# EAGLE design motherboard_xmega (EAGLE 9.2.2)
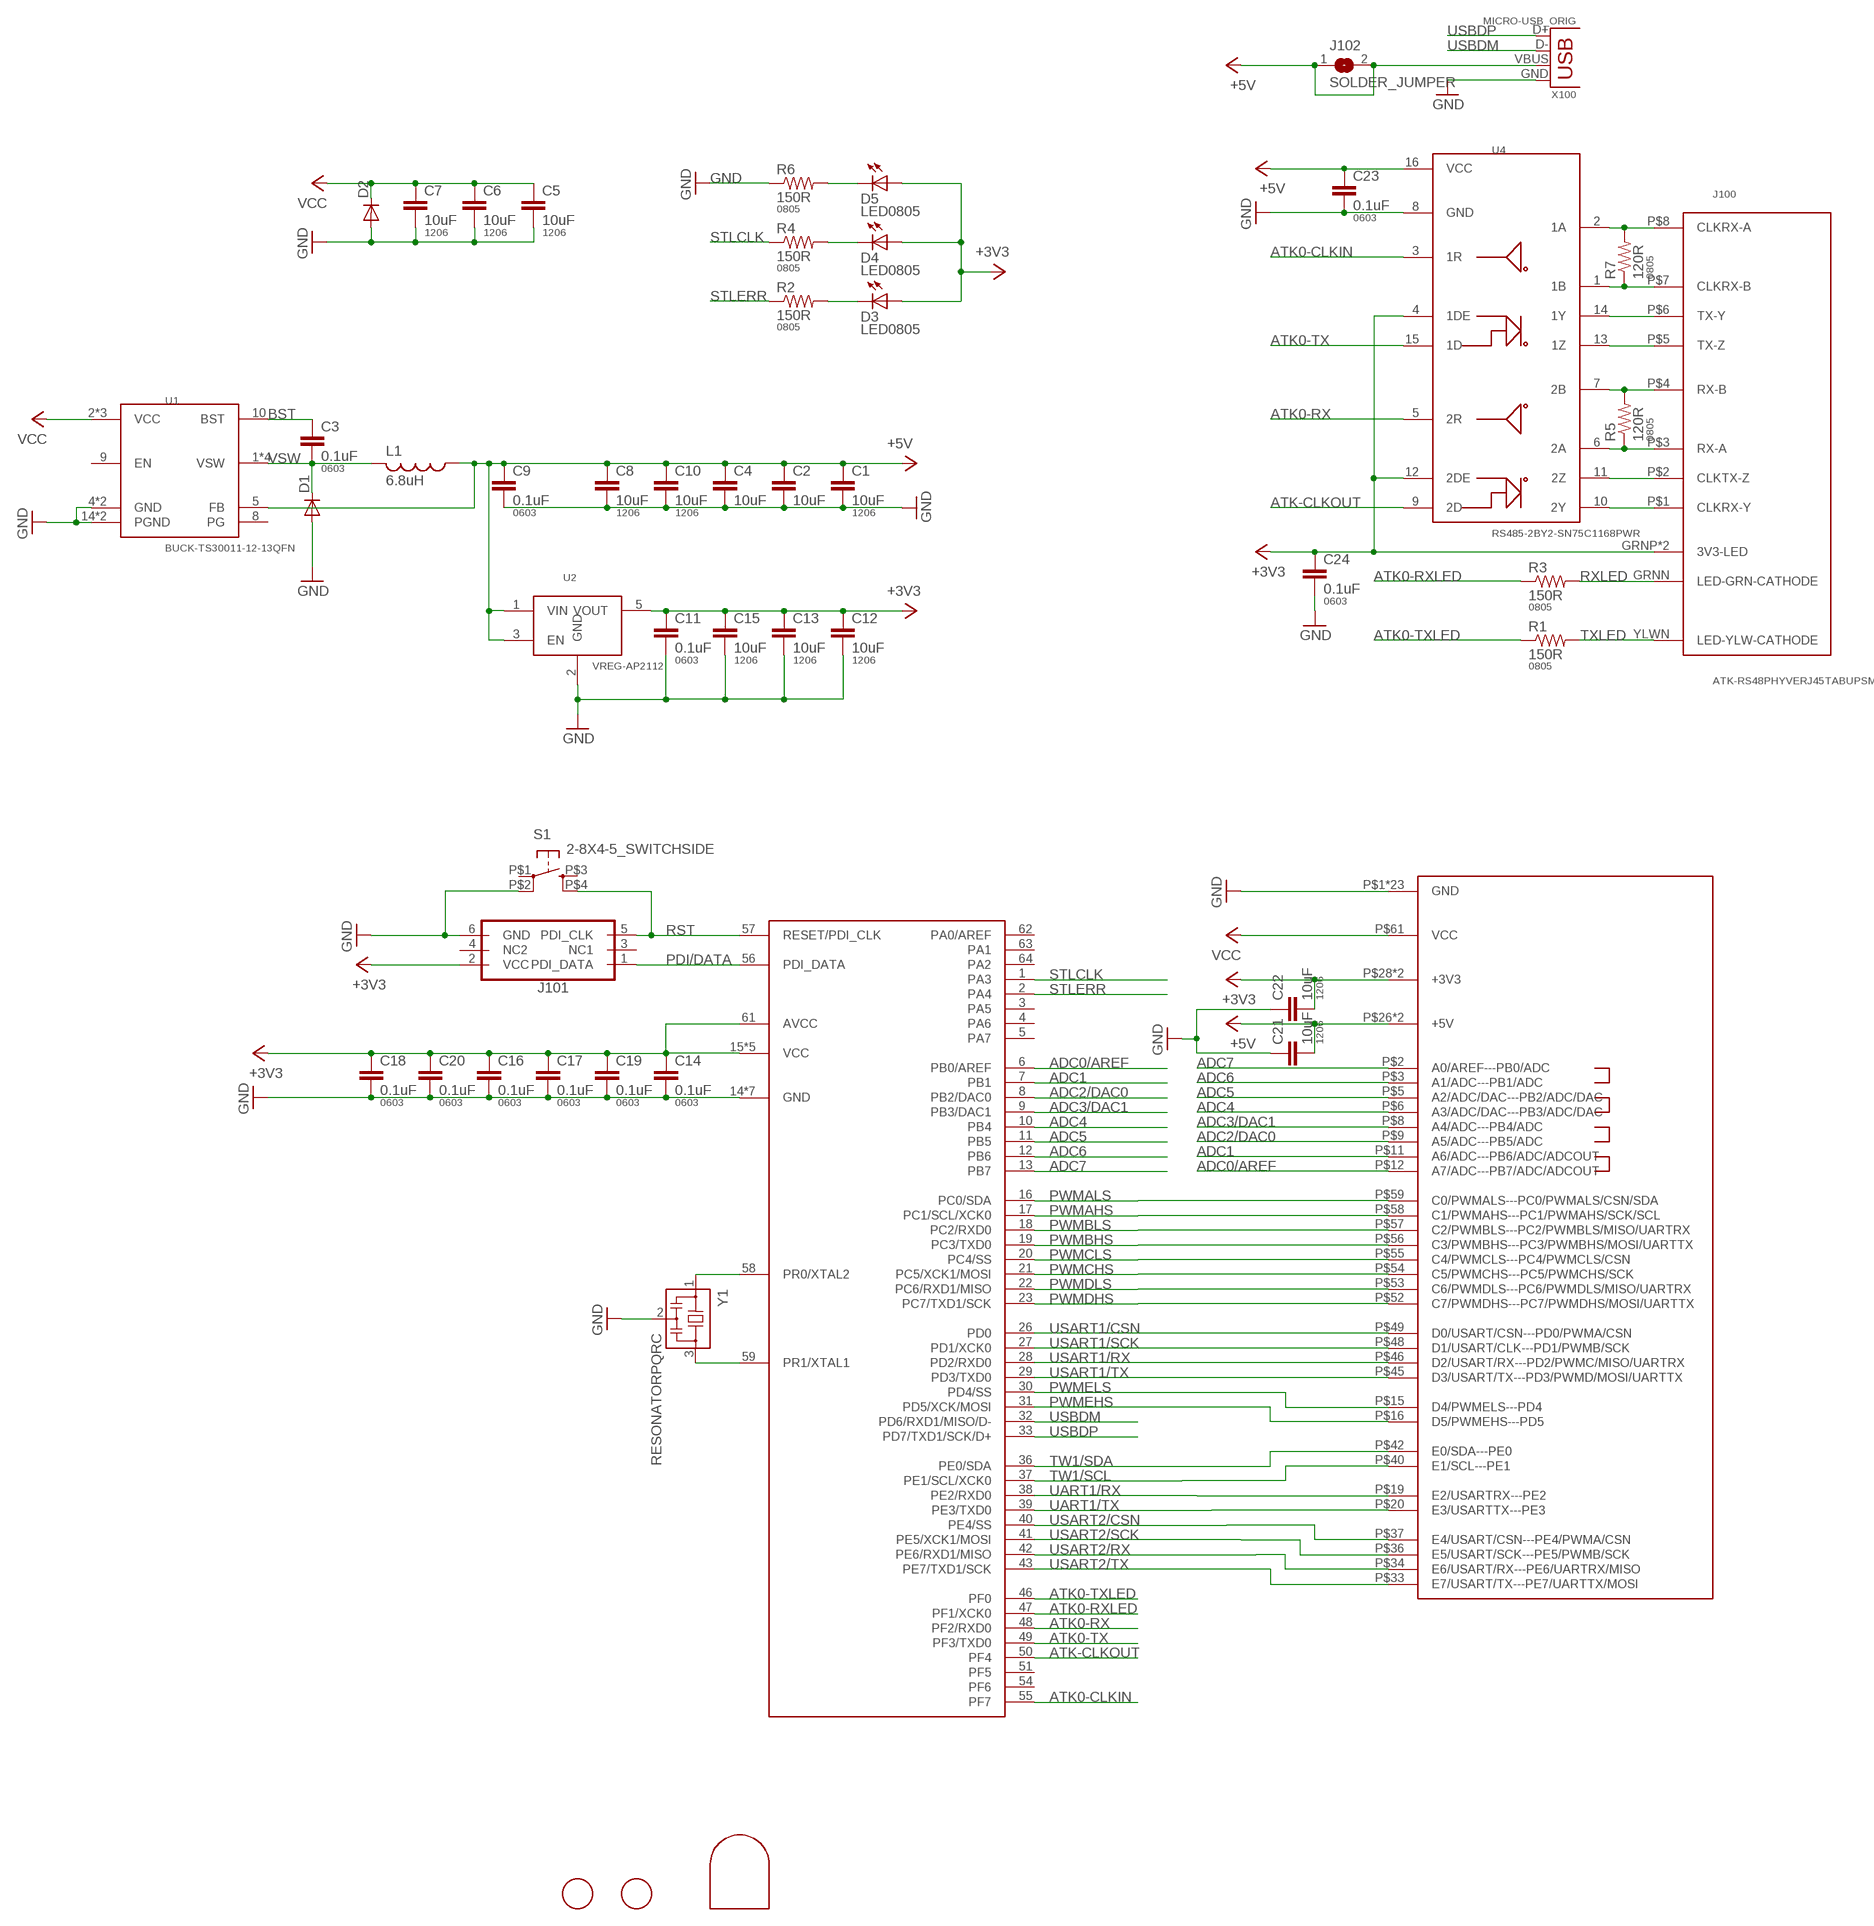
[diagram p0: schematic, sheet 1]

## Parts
C1  10uF  CAP1206  [1206]
C2  10uF  CAP1206  [1206]
C3  0.1uF  CAP0603-CAP  [0603-CAP]
C4  10uF  CAP1206  [1206]
C5  10uF  CAP1206  [1206]
C6  10uF  CAP1206  [1206]
C7  10uF  CAP1206  [1206]
C8  10uF  CAP1206  [1206]
C9  0.1uF  CAP0603-CAP  [0603-CAP]
C10  10uF  CAP1206  [1206]
C11  0.1uF  CAP0603-CAP  [0603-CAP]
C12  10uF  CAP1206  [1206]
C13  10uF  CAP1206  [1206]
C14  0.1uF  CAP0603-CAP  [0603-CAP]
C15  10uF  CAP1206  [1206]
C16  0.1uF  CAP0603-CAP  [0603-CAP]
C17  0.1uF  CAP0603-CAP  [0603-CAP]
C18  0.1uF  CAP0603-CAP  [0603-CAP]
C19  0.1uF  CAP0603-CAP  [0603-CAP]
C20  0.1uF  CAP0603-CAP  [0603-CAP]
C21  10uF  CAP1206  [1206]
C22  10uF  CAP1206  [1206]
C23  0.1uF  CAP0603-CAP  [0603-CAP]
C24  0.1uF  CAP0603-CAP  [0603-CAP]
D1  DIODESOD123HE  [SOD-123HE]
D2  DIODESMA403D  [SMA-403D]
D3  LED0805  [LED0805]
D4  LED0805  [LED0805]
D5  LED0805  [LED0805]
J1  FIDUCIALRCT  [FIDUCIAL_RECT_1MM]
J2  FIDUCIALRCT  [FIDUCIAL_RECT_1MM]
J100  ATK-RS48PHYVERJ45TABUPSMD  [RJ45-LED-SMD-RJWURTH-634008137521]
J101  PDITHRU  [PDI_2X3_THRU]
J102  SOLDER_JUMPER  [SJFAB]
L1  6.8uH  INDUCTOR  [NRS5020T4R7MMGJ]
MP100  JRTOMBSTONE  [JRTOMBSTONE]
R1  150R  RESISTOR0805-RES  [0805]
R2  150R  RESISTOR0805-RES  [0805]
R3  150R  RESISTOR0805-RES  [0805]
R4  150R  RESISTOR0805-RES  [0805]
R5  120R  RESISTOR0805-RES  [0805]
R6  150R  RESISTOR0805-RES  [0805]
R7  120R  RESISTOR0805-RES  [0805]
S1  2-8X4-5_SWITCHSIDE  [TACT-SWITCH-SIDE]
U1  BUCK-TS30011-12-13QFN  [QFN16-3X3-TI-RTE]
U2  VREG-AP2112  [SOT23-5]
U3  ATXMEGA_A3UQFN  [QFN-64-9X9MM]
U4  RS485-2BY2-SN75C1168PWR  [TSSOP16]
U$100  ATK-BFPPFX8-MOTHER  [ATK-BFPP-BOTTOM-FX8-60]
X100  MICRO-USB_ORIG  [DX4R005HJ5]
Y1  RESONATORPQRC  [RES_PRQC]

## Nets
+3V3: C11.1 C12.1 C13.1 C14.1 C15.1 C16.1 C17.1 C18.1 C19.1 C20.1 C22.2 C24.1 D3.1(A) D4.1(A) D5.1(A) J100.GRNP(3V3-LED) J100.YLWP(3V3-LED) J101.2(VCC) U2.5(VOUT) U3.15(VCC) U3.25(VCC) U3.35(VCC) U3.45(VCC) U3.53(VCC) U3.61(AVCC) U4.4(1DE) U4.12(2DE) U$100.P$28(+3V3) U$100.P$29(+3V3)
+5V: C1.1 C2.1 C4.1 C8.1 C9.1 C10.1 C21.2 C23.1 J102.1 J102.2 L1.1 U1.5(FB) U2.1(VIN) U2.3(EN) U4.16(VCC) U$100.P$26(+5V) U$100.P$27(+5V) X100.VBUS
ADC0/AREF: U3.6(PB0/AREF) U$100.P$12(A7/ADC---PB7/ADC/ADCOUT)
ADC1: U3.7(PB1) U$100.P$11(A6/ADC---PB6/ADC/ADCOUT)
ADC2/DAC0: U3.8(PB2/DAC0) U$100.P$9(A5/ADC---PB5/ADC)
ADC3/DAC1: U3.9(PB3/DAC1) U$100.P$8(A4/ADC---PB4/ADC)
ADC4: U3.10(PB4) U$100.P$6(A3/ADC/DAC---PB3/ADC/DAC)
ADC5: U3.11(PB5) U$100.P$5(A2/ADC/DAC---PB2/ADC/DAC)
ADC6: U3.12(PB6) U$100.P$3(A1/ADC---PB1/ADC)
ADC7: U3.13(PB7) U$100.P$2(A0/AREF---PB0/ADC)
ATK0-CLKIN: U3.55(PF7) U4.3(1R)
ATK0-RX: U3.48(PF2/RXD0) U4.5(2R)
ATK0-RXLED: R3.1 U3.47(PF1/XCK0)
ATK0-TX: U3.49(PF3/TXD0) U4.15(1D)
ATK0-TXLED: R1.1 U3.46(PF0)
ATK-CLKOUT: U3.50(PF4) U4.9(2D)
BST: C3.1 U1.10(BST)
GND: C1.2 C2.2 C4.2 C5.2 C6.2 C7.2 C8.2 C9.2 C10.2 C11.2 C12.2 C13.2 C14.2 C15.2 C16.2 C17.2 C18.2 C19.2 C20.2 C21.1 C22.1 C23.2 C24.2 D1.P$2(A) D2.P$2(A) J101.6(GND) R6.1 S1.P$2(P1) U1.4(GND) U1.14(PGND) U1.15(PGND) U1.TH(GND) U2.2(GND) U3.14(GND) U3.24(GND) U3.34(GND) U3.44(GND) U3.52(GND) U3.60(GND) U3.P$1(GND) U4.8(GND) U$100.P$1(GND) U$100.P$4(GND) U$100.P$7(GND) U$100.P$10(GND) U$100.P$13(GND) U$100.P$14(GND) U$100.P$17(GND) U$100.P$18(GND) U$100.P$21(GND) U$100.P$30(GND) U$100.P$31(GND) U$100.P$32(GND) U$100.P$35(GND) U$100.P$38(GND) U$100.P$39(GND) U$100.P$41(GND) U$100.P$43(GND) U$100.P$44(GND) U$100.P$47(GND) U$100.P$50(GND) U$100.P$51(GND) U$100.P$60(GND) U$100.P$62(GND) X100.GND Y1.2
N$1: U3.58(PR0/XTAL2) Y1.1
N$2: U3.59(PR1/XTAL1) Y1.3
N$8: J100.P$8(CLKRX-A) R7.2 U4.2(1A)
N$9: D5.2(C) R6.2
N$10: D4.2(C) R4.2
N$11: D3.2(C) R2.2
N$12: J100.P$7(CLKRX-B) R7.1 U4.1(1B)
N$13: J100.P$6(TX-Y) U4.14(1Y)
N$14: J100.P$5(TX-Z) U4.13(1Z)
N$15: J100.P$4(RX-B) R5.2 U4.7(2B)
N$16: J100.P$3(RX-A) R5.1 U4.6(2A)
N$17: J100.P$2(CLKTX-Z) U4.11(2Z)
N$18: J100.P$1(CLKRX-Y) U4.10(2Y)
PDI/DATA: J101.1(PDI_DATA) U3.56(PDI_DATA)
PWMAHS: U3.17(PC1/SCL/XCK0) U$100.P$58(C1/PWMAHS---PC1/PWMAHS/SCK/SCL)
PWMALS: U3.16(PC0/SDA) U$100.P$59(C0/PWMALS---PC0/PWMALS/CSN/SDA)
PWMBHS: U3.19(PC3/TXD0) U$100.P$56(C3/PWMBHS---PC3/PWMBHS/MOSI/UARTTX)
PWMBLS: U3.18(PC2/RXD0) U$100.P$57(C2/PWMBLS---PC2/PWMBLS/MISO/UARTRX)
PWMCHS: U3.21(PC5/XCK1/MOSI) U$100.P$54(C5/PWMCHS---PC5/PWMCHS/SCK)
PWMCLS: U3.20(PC4/SS) U$100.P$55(C4/PWMCLS---PC4/PWMCLS/CSN)
PWMDHS: U3.23(PC7/TXD1/SCK) U$100.P$52(C7/PWMDHS---PC7/PWMDHS/MOSI/UARTTX)
PWMDLS: U3.22(PC6/RXD1/MISO) U$100.P$53(C6/PWMDLS---PC6/PWMDLS/MISO/UARTRX)
PWMEHS: U3.31(PD5/XCK/MOSI) U$100.P$16(D5/PWMEHS---PD5)
PWMELS: U3.30(PD4/SS) U$100.P$15(D4/PWMELS---PD4)
RST: J101.5(PDI_CLK) S1.P$4(S1) U3.57(RESET/PDI_CLK)
RXLED: J100.GRNN(LED-GRN-CATHODE) R3.2
STLCLK: R4.1 U3.1(PA3)
STLERR: R2.1 U3.2(PA4)
TW1/SCL: U3.37(PE1/SCL/XCK0) U$100.P$40(E1/SCL---PE1)
TW1/SDA: U3.36(PE0/SDA) U$100.P$42(E0/SDA---PE0)
TXLED: J100.YLWN(LED-YLW-CATHODE) R1.2
UART1/RX: U3.38(PE2/RXD0) U$100.P$19(E2/USARTRX---PE2)
UART1/TX: U3.39(PE3/TXD0) U$100.P$20(E3/USARTTX---PE3)
USART1/CSN: U3.26(PD0) U$100.P$49(D0/USART/CSN---PD0/PWMA/CSN)
USART1/RX: U3.28(PD2/RXD0) U$100.P$46(D2/USART/RX---PD2/PWMC/MISO/UARTRX)
USART1/SCK: U3.27(PD1/XCK0) U$100.P$48(D1/USART/CLK---PD1/PWMB/SCK)
USART1/TX: U3.29(PD3/TXD0) U$100.P$45(D3/USART/TX---PD3/PWMD/MOSI/UARTTX)
USART2/CSN: U3.40(PE4/SS) U$100.P$37(E4/USART/CSN---PE4/PWMA/CSN)
USART2/RX: U3.42(PE6/RXD1/MISO) U$100.P$34(E6/USART/RX---PE6/UARTRX/MISO)
USART2/SCK: U3.41(PE5/XCK1/MOSI) U$100.P$36(E5/USART/SCK---PE5/PWMB/SCK)
USART2/TX: U3.43(PE7/TXD1/SCK) U$100.P$33(E7/USART/TX---PE7/UARTTX/MOSI)
USBDM: U3.32(PD6/RXD1/MISO/D-) X100.D-
USBDP: U3.33(PD7/TXD1/SCK/D+) X100.D+
VCC: C5.1 C6.1 C7.1 D2.P$1(C) U1.2(VCC) U1.3(VCC) U1.11(VCC) U$100.P$61(VCC)
VSW: C3.2 D1.P$1(C) L1.2 U1.1(VSW) U1.12(VSW) U1.13(VSW) U1.16(VSW)
Unconnected: J101.3(NC1) J101.4(NC2) S1.P$1(P) S1.P$3(S) U1.8(PG) U1.9(EN) U3.3(PA5) U3.4(PA6) U3.5(PA7) U3.51(PF5) U3.54(PF6) U3.62(PA0/AREF) U3.63(PA1) U3.64(PA2)

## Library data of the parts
C1 C2 C4-C8 C10 C12 C13 C15 C21 C22 = passives:CAP: Capacitor; PACKAGE: 1206
C3 C9 C11 C14 C16-C20 C23 C24 = passives:CAP: Capacitor; PACKAGE: 0603
D1 D2 = passives:DIODE: DIODE
D3-D5 = lights:LED: LED
J1 J2 = connector:FIDUCIAL: For use by pick and place machines to calibrate the vision/machine, 1mm
J100 = connector:ATK-RS48PHYVE
J101 = microcontrollers:PDI: Multi connection point. Often used as Generic Header-pin footprint for 0.1 inch spaced/style header connections You can populate with any combo of single row headers, but if you'd like an exact match, check these: Header - 2x3 (Male, 0.1") (PRT-12807) Header - 2x3 (Female, 0.1") (PRT-13010) 2x3 Pin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
J102 = connector:SOLDER_JUMPER
L1 = power:INDUCTOR
MP100 = connector:JRTOMBSTONE
R1-R7 = borkedlabs-passives:RESISTOR: Resistor; PACKAGE: 0805
S1 = passives:2-8X4-5_SWITCH
U1 = power:BUCK-TS30011-12-13
U2 = power:VREG-AP2112
U3 = microcontrollers:ATXMEGA_A3U
U4 = comm:RS485-2BY2-SN75C1168PWR
U$100 = connector:ATK-BFPP
X100 = connector:MICRO-USB: SMD micro USB connector as found in the fablab inventory. Three footprint variants included: original, as described by manufacturer's datasheet for milling with the 1/100" bit for milling with the 1/64" bit Made by Zaerc.
Y1 = passives:RESONATOR

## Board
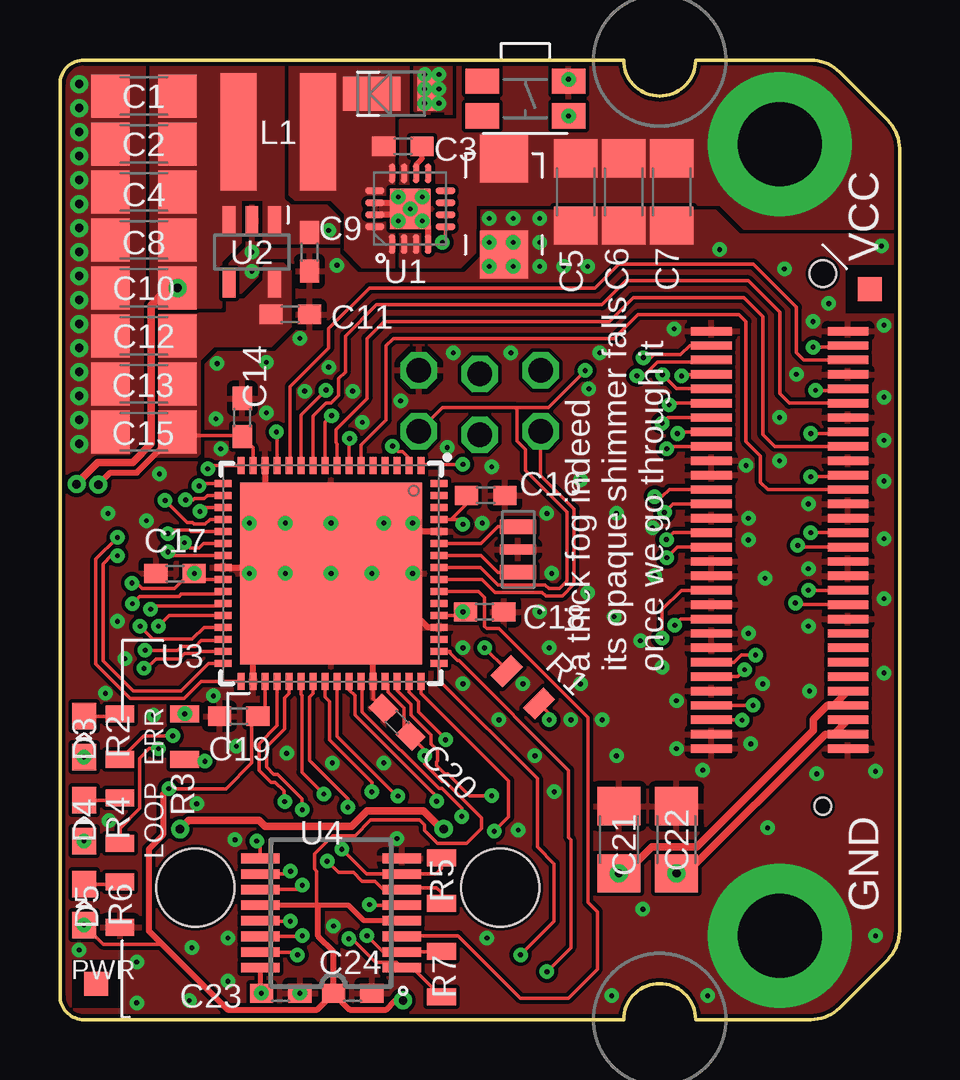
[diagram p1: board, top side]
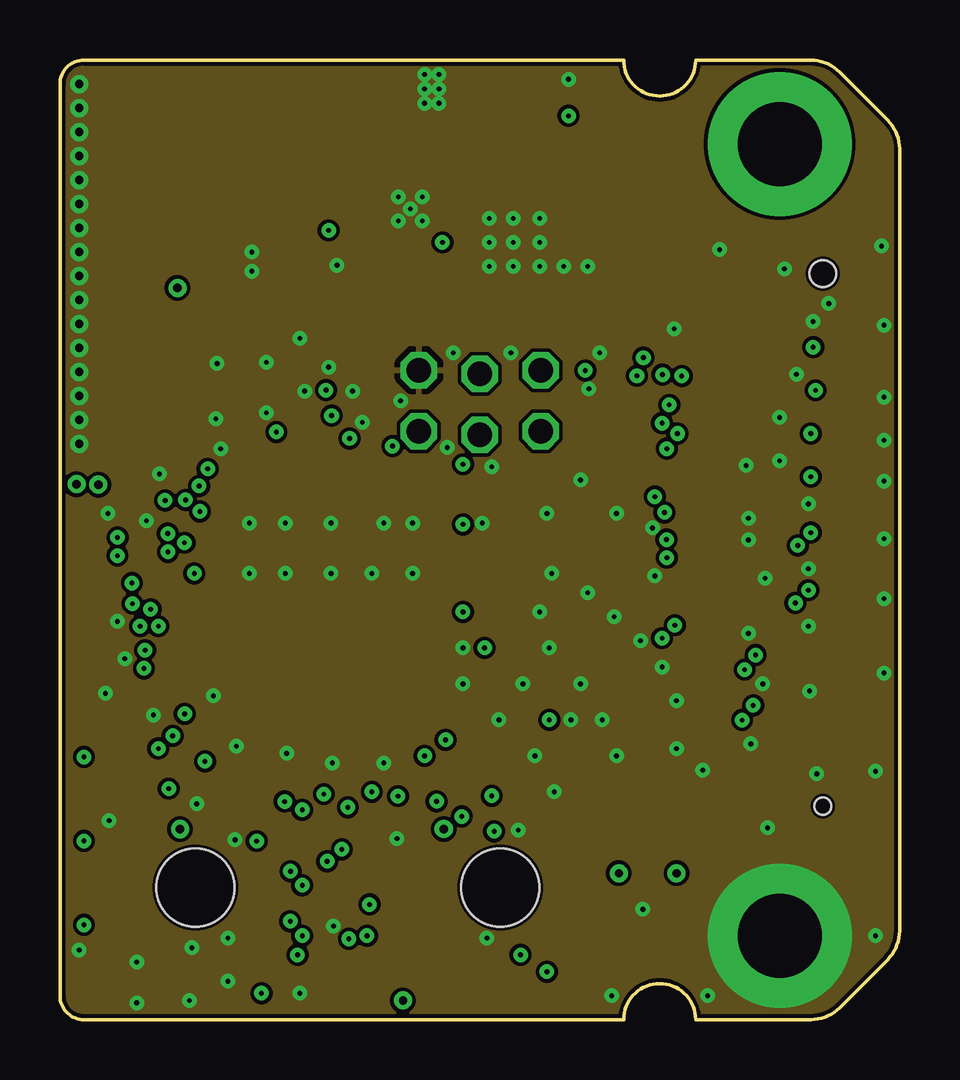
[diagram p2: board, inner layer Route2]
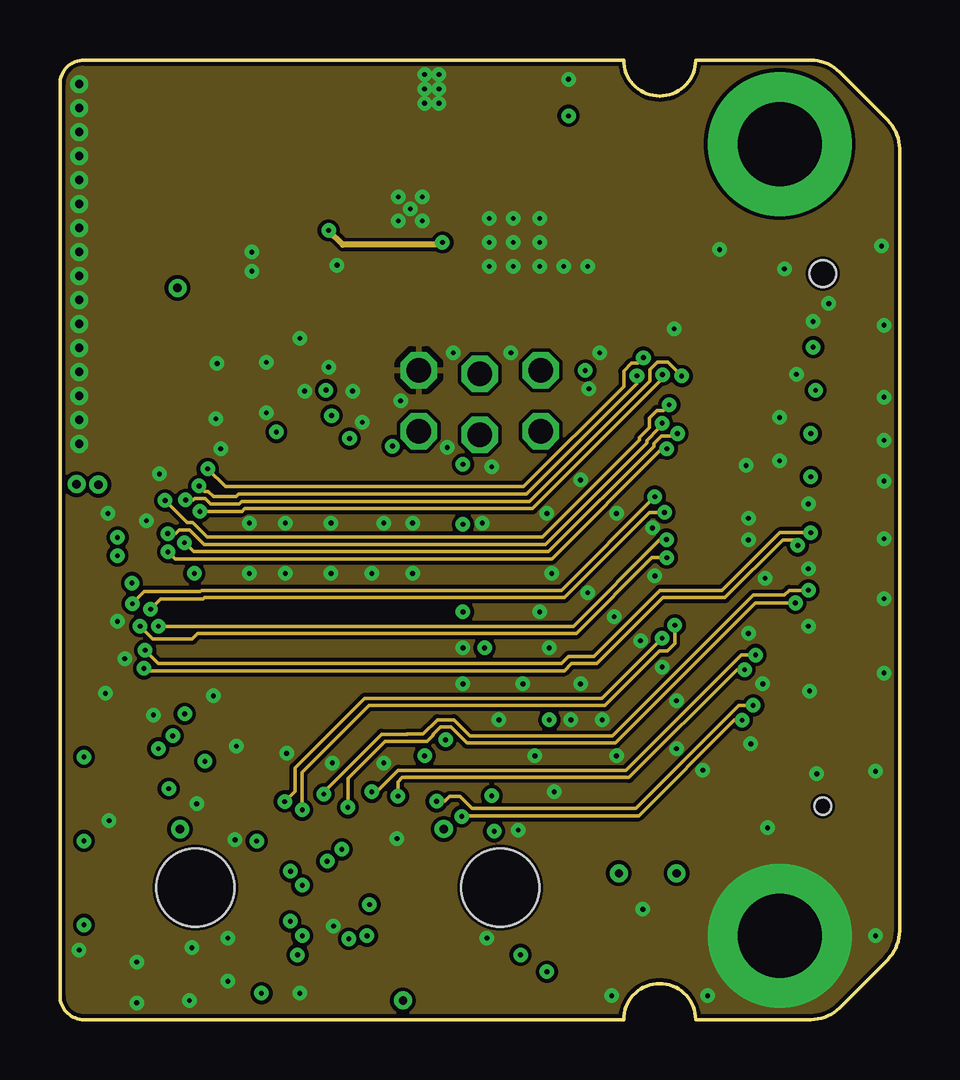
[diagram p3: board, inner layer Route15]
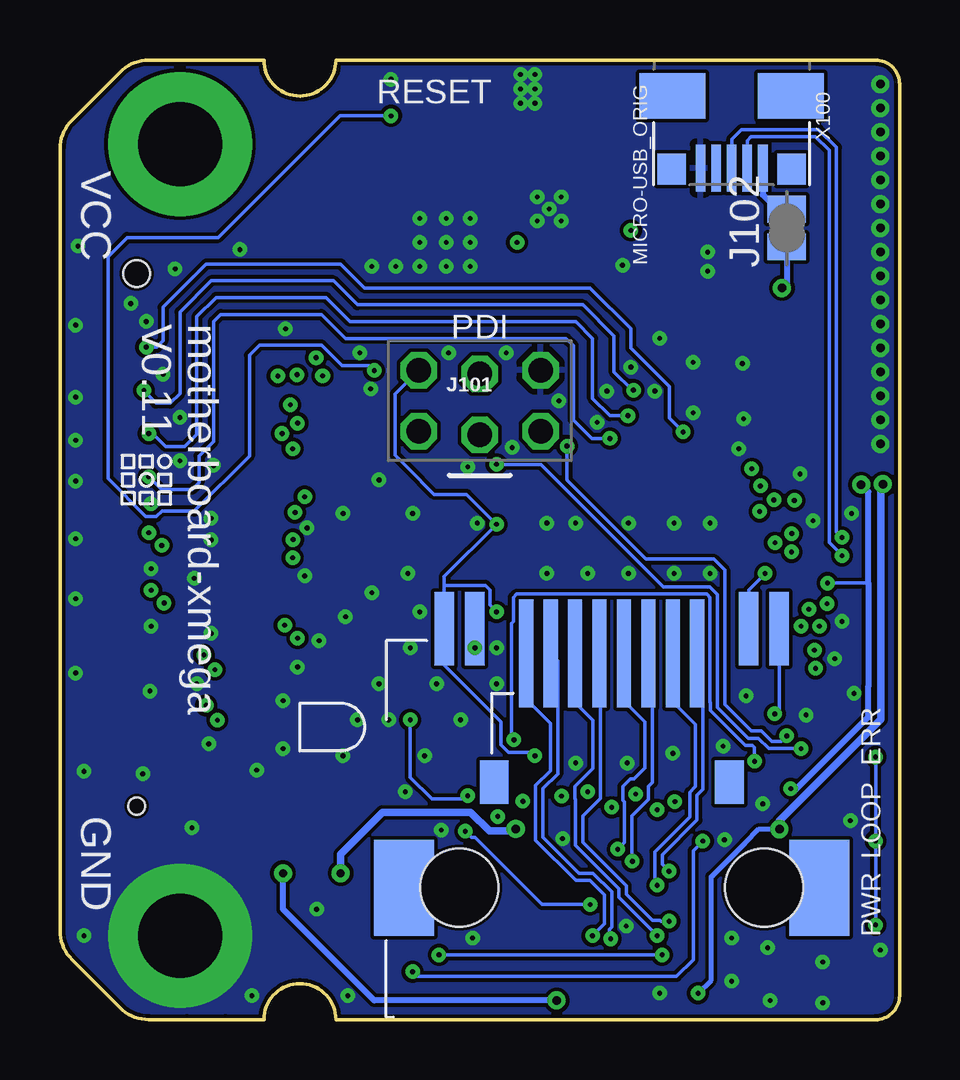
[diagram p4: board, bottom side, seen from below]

Size 35 x 40.01 mm. Coordinates in mm from the lower left corner, seen from the top.
Outline: 23.5,40 arc90 25,38.5 arc90 26.5,40 arc0 31.3,40 arc-45 32.5,39.5 34.5,37.5 arc-45 35,36.3 35,3.7 arc-45 34.5,2.5 32.5,0.5 arc-45 31.3,0 arc0 26.5,0 arc90 25,1.5 arc90 23.5,0 1,0 arc-90 0,1 0,39 arc-90 1,40 23.5,40
Copper layers (1+2*15+16): Top 0.035mm / dielectric 0.3mm / Route2 0.035mm / dielectric 0.3mm / Route15 0.035mm / dielectric 0.3mm / Bottom 0.035mm
Design rules "default *": minimum track width 6mil, minimum drill 0.2mm, track to track 6mil, track to pad 6mil, pad to pad 6mil, via to via 6mil, smd to smd 6mil, copper to edge 6mil, drill to drill 6mil, minimum pad ring 10mil, minimum via ring 8mil, stop-mask expansion 4mil, vias tented up to drill 25mil, thermal gap 10mil

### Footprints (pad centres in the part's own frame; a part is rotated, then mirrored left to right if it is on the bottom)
1206 = smd 1.6 x 1.8: 1 -1.4,0; 2 1.4,0
0603-CAP = smd 0.96 x 0.8: 1 -0.8,0; 2 0.8,0
SOD-123HE = smd 2.4 x 1.4: P$1 0.8,0 | smd 0.9 x 1.4: P$2 -1.55,0
SMA-403D = smd 2 x 2: P$1 -2,0; P$2 2,0
LED0805 = smd 1.1 x 1: 1 -0.85,0; 2 0.85,0
FIDUCIAL_RECT_1MM = smd 1 x 1: P$1 0,0
RJ45-LED-SMD-RJWURTH-634008137521 = smd 0.8 x 3.05: GRNN 6.98,10.8; GRNP 5.71,10.8; YLWN -5.71,10.8; YLWP -6.98,10.8 | smd 0.6 x 4.5: P$1 3.57,9.76; P$2 2.55,9.76; P$3 1.53,9.76; P$4 0.51,9.76; P$5 -0.51,9.76; P$6 -1.53,9.76; P$7 -2.55,9.76; P$8 -3.57,9.76 | smd 1.2 x 1.8: P$9 -4.9,4.4; P$10 4.9,4.4 | smd 2.5 x 4: P$13 -8.65,0; P$14 8.65,0 | hole 3.25: -6.35,0; 6.35,0
PDI_2X3_THRU = drill 1.016 octagon: 1 -2.54,-1.27; 2 -2.54,1.27; 3 0,-1.42; 4 0,1.12; 5 2.54,-1.27; 6 2.54,1.27
SJFAB = smd 1.118 x 1.6: 1 -0.787,0; 2 0.787,0
NRS5020T4R7MMGJ = smd 4.9 x 1.5: 1 0,1.65; 2 0,-1.65
0805 = smd 0.7 x 1.2: 1 -0.95,0; 2 0.95,0
TACT-SWITCH-SIDE = smd 1.4 x 1.05: P$1 -1.8,0.725; P$2 1.8,0.725; P$3 -1.8,-0.725; P$4 1.8,-0.725
QFN16-3X3-TI-RTE = smd 0.8 x 0.275: 1 -1.475,0.75; 2 -1.475,0.25; 3 -1.475,-0.25; 4 -1.475,-0.75; 9 1.475,-0.75; 10 1.475,-0.25; 11 1.475,0.25; 12 1.475,0.75 | smd 0.275 x 0.8: 5 -0.75,-1.475; 6 -0.25,-1.475; 7 0.25,-1.475; 8 0.75,-1.475; 13 0.75,1.475; 14 0.25,1.475; 15 -0.25,1.475; 16 -0.75,1.475 | smd 1.7 x 1.7: TH 0,0
SOT23-5 = smd 0.533 x 1.194: 1 -0.95,-1.306; 2 0,-1.306; 3 0.95,-1.306; 4 0.95,1.306; 5 -0.95,1.306
QFN-64-9X9MM = smd 0.7 x 0.275: 1 -4.5,3.75; 2 -4.5,3.25; 3 -4.5,2.75; 4 -4.5,2.25; 5 -4.5,1.75; 6 -4.5,1.25; 7 -4.5,0.75; 8 -4.5,0.25; 9 -4.5,-0.25; 10 -4.5,-0.75; 11 -4.5,-1.25; 12 -4.5,-1.75; 13 -4.5,-2.25; 14 -4.5,-2.75; 15 -4.5,-3.25; 16 -4.5,-3.75; 33 4.5,-3.75; 34 4.5,-3.25; 35 4.5,-2.75; 36 4.5,-2.25; 37 4.5,-1.75; 38 4.5,-1.25; 39 4.5,-0.75; 40 4.5,-0.25; 41 4.5,0.25; 42 4.5,0.75; 43 4.5,1.25; 44 4.5,1.75; 45 4.5,2.25; 46 4.5,2.75; 47 4.5,3.25; 48 4.5,3.75 | smd 0.275 x 0.7: 17 -3.75,-4.5; 18 -3.25,-4.5; 19 -2.75,-4.5; 20 -2.25,-4.5; 21 -1.75,-4.5; 22 -1.25,-4.5; 23 -0.75,-4.5; 24 -0.25,-4.5; 25 0.25,-4.5; 26 0.75,-4.5; 27 1.25,-4.5; 28 1.75,-4.5; 29 2.25,-4.5; 30 2.75,-4.5; 31 3.25,-4.5; 32 3.75,-4.5; 49 3.75,4.5; 50 3.25,4.5; 51 2.75,4.5; 52 2.25,4.5; 53 1.75,4.5; 54 1.25,4.5; 55 0.75,4.5; 56 0.25,4.5; 57 -0.25,4.5; 58 -0.75,4.5; 59 -1.25,4.5; 60 -1.75,4.5; 61 -2.25,4.5; 62 -2.75,4.5; 63 -3.25,4.5; 64 -3.75,4.5 | smd 7.6 x 7.6: P$1 0,0
TSSOP16 = smd 0.4 x 1.6: 1 -2.225,-2.85; 2 -1.575,-2.85; 3 -0.925,-2.85; 4 -0.275,-2.85; 5 0.375,-2.85; 6 1.025,-2.85; 7 1.675,-2.85; 8 2.325,-2.85; 9 2.325,3.05; 10 1.675,3.05; 11 1.025,3.05; 12 0.375,3.05; 13 -0.275,3.05; 14 -0.925,3.05; 15 -1.575,3.05; 16 -2.225,3.05
ATK-BFPP-BOTTOM-FX8-60 = smd 0.35 x 1.7 bottom: P$1 -8.7,-2.85; P$2 -8.1,-2.85; P$3 -7.5,-2.85; P$4 -6.9,-2.85; P$5 -6.3,-2.85; P$6 -5.7,-2.85; P$7 -5.1,-2.85; P$8 -4.5,-2.85; P$9 -3.9,-2.85; P$10 -3.3,-2.85; P$11 -2.7,-2.85; P$12 -2.1,-2.85; P$13 -1.5,-2.85; P$14 -0.9,-2.85; P$15 -0.3,-2.85; P$16 0.3,-2.85; P$17 0.9,-2.85; P$18 1.5,-2.85; P$19 2.1,-2.85; P$20 2.7,-2.85; P$21 3.3,-2.85; P$22 3.9,-2.85; P$23 4.5,-2.85; P$24 5.1,-2.85; P$25 5.7,-2.85; P$26 6.3,-2.85; P$27 6.9,-2.85; P$28 7.5,-2.85; P$29 8.1,-2.85; P$30 8.7,-2.85; P$31 8.7,2.85; P$32 8.1,2.85; P$33 7.5,2.85; P$34 6.9,2.85; P$35 6.3,2.85; P$36 5.7,2.85; P$37 5.1,2.85; P$38 4.5,2.85; P$39 3.9,2.85; P$40 3.3,2.85; P$41 2.7,2.85; P$42 2.1,2.85; P$43 1.5,2.85; P$44 0.9,2.85; P$45 0.3,2.85; P$46 -0.3,2.85; P$47 -0.9,2.85; P$48 -1.5,2.85; P$49 -2.1,2.85; P$50 -2.7,2.85; P$51 -3.3,2.85; P$52 -3.9,2.85; P$53 -4.5,2.85; P$54 -5.1,2.85; P$55 -5.7,2.85; P$56 -6.3,2.85; P$57 -6.9,2.85; P$58 -7.5,2.85; P$59 -8.1,2.85; P$60 -8.7,2.85 | drill 3.5 pad 6: P$61 -16.5,0; P$62 16.5,0 | hole 1.1: -11.1,-1.8 | hole 0.7: 11.1,-1.8
DX4R005HJ5 = smd 0.4 x 1.95: D+ 0,1.9; D- -0.65,1.9; GND 1.3,1.9; ID 0.65,1.9; VBUS -1.3,1.9 | smd 1.2 x 1.3: GND@1 -2.5,1.95; GND@2 2.5,1.95 | smd 2.75 x 1.9: GND@3 -2.475,-1.1; GND@4 2.475,-1.1
RES_PRQC = smd 0.6 x 1.5: 1 -0.95,0; 3 0.95,0 | smd 0.4 x 1.5: 2 0,0

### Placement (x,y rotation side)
C1  3.5,38.5 180 top
C2  3.5,36.5 180 top
C3  14.3,36.4 180 top
C4  3.5,34.5 180 top
C5  21.5,34.5 270 top
C6  23.5,34.5 270 top
C7  25.5,34.5 270 top
C8  3.5,32.5 180 top
C9  10.4,32 270 top
C10  3.5,30.5 180 top
C11  9.6,29.4 0 top
C12  3.5,28.5 180 top
C13  3.5,26.5 180 top
C14  7.6,25.1 90 top
C15  3.5,24.5 180 top
C16  17.75,21.85 0 top
C17  4.8,18.6 180 top
C18  17.7,17 0 top
C19  7.45,12.65 180 top
C20  14.05,12.4 135 top
C21  23.3,7.5 270 top
C22  25.7,7.5 270 top
C23  9.2,1.1 0 top
C24  12.2,1.1 0 top
D1  13.8,38.6 180 top
D2  18.5,33.9 270 top
D3  1,11.8 90 top
D4  1,8.3 90 top
D5  1,4.8 90 top
J1  33.75,30.45 90 top
J2  1.5,1.5 0 top
J100  12,5.5 0 bottom
J101  17.5,25.8 0 bottom
J102  4.7,33 90 bottom
L1  9.1,37 90 top
MP100  24,12.2 270 bottom
R1  19.3,13.85 135 top
R2  2.5,11.8 90 top
R3  5.2,11.8 90 top
R4  2.5,8.3 90 top
R5  15.9,5.8 90 top
R6  2.5,4.8 90 top
R7  15.9,1.9 90 top
S1  19.4,38.4 0 top
U1  14.6,33.8 90 top
U2  8,32 180 top
U3  11.3,18.6 270 top
U4  11.4,4.4 90 top
U$100  30,20 270 bottom
U$101  CBA-LOGO  [CBA-SILK-LOGO]  31.4,22.5 270 bottom
X100  7,37.4 180 bottom
Y1  19.1,19.6 90 top

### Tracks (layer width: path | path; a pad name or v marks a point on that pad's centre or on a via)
+3V3  (via drill 0.2, 0.35)
  Top 0.152: U3.45 13.68,13.97 13.68,13.66 14.34,13.01 14.34,12.12 C20.1 15.2,11.25 v15.2,11 15.2,10.67 15.93,9.94 16.05,9.94 17.58,8.41 17.58,7.98 16.95,7.35 15.75,7.35 15.19,7.9 15.19,8.12 14.99,8.32 12.96,8.32 12.31,7.67 11.36,7.67 10.61,6.92 10.61,6.28 10.7,6.19 10.7,4.78 10.77,4.71 | U3.35 8.55,12.95 C19.1 8,12.4 8,10.7 6.92,9.63 v4.53,9.63 | U3.53 16.65,16.85 v16.8,17 C18.1 | U3.25 5.85,18.35 C17.1 5.4,18.6 4.77,17.98 3.43,17.98 3.2,18.2 v3,18.2 | U3.15 8.05,23.85 C14.1 7.55,24.35 5.05,24.35 C15.1 | U3.61 16.3,20.85 | 16.3,20.85 16.95,21.5 C16.1 | 16.3,20.85 16.6,20.85 v16.8,20.65 | D5.1 1.8,3.15 4.25,3.15
  Top 0.203: U4.4 12.68,4.13 12.03,4.78 10.7,4.78 U4.12
  Top 0.254: v1.6,22.3 2.1,22.8 3.2,22.8 C15.1 | C24.1 11.4,2.85 10.77,3.48 10.77,4.71 | v4.53,9.63 4.3,9.4 4.3,7.7 3.7,7.1 3.7,3.7 4.25,3.15 6.98,0.43 10.72,0.43 C24.1 | v14.3,0.8 13.97,0.8 13.6,0.43 12.08,0.43 C24.1
  Top 0.305: U$100.P$29 32.25,11.9 | 32.25,11.9 31.9,11.9 26.1,6.1 C22.2 | U$100.P$28 32.25,11.9
  Bottom 0.152: D5.1 D4.1 D3.1 | v3,18.2 1.3,18.2 | 18.98,18.1 18.98,18.47 v16.8,20.65 17.07,20.92 18.05,21.9 19.4,21.9 20.5,23 20.55,23.05 21.03,23.54 21.03,26.08 J101.2 | 18.98,18.1 J100.YLWP 18.98,14.78 16.61,12.41 16.61,11.45 16.3,11.14 15.33,11.14 v15.2,11 | J100.GRNP 6.29,17.91 C17.1 | v16.8,17 17.08,17.29 17.08,17.92 17.26,18.1 18.98,18.1
  Bottom 0.254: v1.6,22.3 1.3,22 1.3,18.2 1.3,13.9 1.32,13.89 1.32,12.6 4.41,9.51 v4.53,9.63 | v14.3,0.8 21.9,0.8 25.7,4.6 C22.2
  other vias: 1,10.95 1,7.45 1,3.95 25.7,6.1 5.6,18.6
  pour Top (rank 4, no thermals): 9.6,28.9 9.6,31.2 9.3,31.5 8.6,31.5 8.5,31.4 8.5,30.8 7.7,30 3.7,30 3.7,23.8 4,23.5 5.7,23.5 5.8,23.6 5.8,27.5 6.4,28.1 8.8,28.1
+5V  (via drill 0.2, 0.35)
  Top 0.152: U1.5 16.07,32.54 v15.94,32.4
  Top 0.203: U4.16 8.35,1.15 C23.1
  Top 0.305: C10.1 4.7,30.3 4.3,30.3 3.8,29.8 3.8,24.01 3.02,23.24 1.57,23.24 0.92,22.59 0.92,22.55 v0.69,22.33 | U$100.P$27 32.25,13.1 | C21.2 23.57,6.1 24.67,7.21 26.56,7.21 31.4,12.05 31.4,12.51 31.99,13.1 32.25,13.1 | U$100.P$26 32.25,13.1 | v16,7.95 15.9,7.95 15.15,8.7 12.8,8.7 12.15,8.05 8.55,8.05 8.3,8.3 5.37,8.3 v5.01,7.95
  Route15 0.254: v15.94,32.4 15.84,32.3 11.8,32.3 v11.2,32.9
  Bottom 0.152: X100.VBUS 5.7,35.6
  Bottom 0.203: C23.1 7.85,1.65 7.85,5.96 6.43,7.38 6.42,7.38 5.86,7.95 v5.01,7.95
  Bottom 0.254: 5.7,35.6 5.7,34.39 5.1,33.79 J102.2 J102.1 4.7,30.7 C10.1
  Bottom 0.305: v0.69,22.33 0.79,22.23 0.79,12.51 5.01,8.3 v5.01,7.95 | v16,7.95 16.09,7.86 17.1,7.86 17.89,8.65 21.55,8.65 23.3,6.9 C21.2
  other vias: 4.9,30.5 8.4,1.1 23.3,6.1
  pour Top (rank 3, no thermals): 11.7,32.4 8.5,32.4 8.5,34.2 7.5,34.2 7.5,32.4 6.7,31.6 6.7,29.7 3.7,29.7 3.7,40.5 9.4,40.5 9.4,34.4 9.8,34 11.3,34 11.7,33.6
ADC0/AREF
  Top 0.152: U$100.P$12 29.5,22.1 29.2,22.4 29.2,23.5 28.6,24.1 28.6,29.1 28.3,29.4 24.1,29.4 23.1,28.4 13.9,28.4 13.6,28.1 13.6,25 12.55,23.95 U3.6
ADC1  (via drill 0.2)
  Top 0.152: U3.7 12.05,24.21 v12.07,24.23 | v31.3,22.64 32.78,22.64 U$100.P$11
  Bottom 0.152: v12.07,24.23 12.83,24.23 13.6,25 13.6,28.1 13.9,28.4 23.1,28.4 24.1,29.4 28.3,29.4 28.6,29.1 28.6,24.1 29.2,23.5 29.2,22.4 29.5,22.1 30.77,22.1 v31.3,22.64
ADC2/DAC0
  Top 0.152: U$100.P$9 29.8,23.9 29.3,24.4 29.3,29.3 28.5,30.1 23.9,30.1 22.9,29.1 13.5,29.1 12.8,28.4 12.8,25.9 11.5,24.6 11.5,24.05 11.55,24 U3.8
ADC3/DAC1  (via drill 0.2)
  Top 0.152: U3.9 11.05,24.91 v11.32,25.18 | v31.3,24.44 32.78,24.44 U$100.P$8
  Bottom 0.152: v11.32,25.18 12.08,25.18 12.8,25.9 12.8,28.4 13.5,29.1 22.9,29.1 23.9,30.1 28.5,30.1 29.3,29.3 29.3,24.4 29.8,23.9 30.6,23.9 31.13,24.44 v31.3,24.44
ADC4
  Top 0.152: U$100.P$6 30.4,25.7 30,26.1 30,29.5 28.7,30.8 23.6,30.8 22.6,29.8 13.2,29.8 11.9,28.5 11.9,27 11.62,26.72 11.62,26.02 11.31,25.71 11.1,25.71 10.55,25.16 U3.10
ADC5  (via drill 0.2)
  Top 0.152: U3.11 10.05,25.21 v11.09,26.24 | v31.5,26.24 32.78,26.24 U$100.P$5
  Bottom 0.152: v11.09,26.24 11.14,26.24 11.9,27 11.9,28.5 13.2,29.8 22.6,29.8 23.6,30.8 28.7,30.8 30,29.5 30,26.1 30.4,25.7 31,25.7 31.5,26.2 v31.5,26.24
ADC6
  Top 0.152: U$100.P$3 31,27.5 30.7,27.8 30.7,29.7 28.9,31.5 23.3,31.5 22.3,30.5 12.9,30.5 11.2,28.8 11.2,28 9.6,26.4 9.6,23.15 U3.12
ADC7  (via drill 0.2)
  Top 0.152: U3.13 9.05,24.47 v9.02,24.5 | v31.4,28.04 32.78,28.04 U$100.P$2
  Bottom 0.152: v9.02,24.5 9.6,25.09 9.6,26.4 11.2,28 11.2,28.8 12.9,30.5 22.3,30.5 23.3,31.5 28.9,31.5 30.7,29.7 30.7,28.3 30.97,28.04 v31.4,28.04
ATK0-CLKIN
  Top 0.152: U3.55 17.45,17.85 17.7,17.6 17.7,16.4 17.8,16.3 18.3,16.3 22,12.6 22,4.9 22.4,4.5 22.4,2.1 21.2,0.9 19.2,0.9 16.6,3.5 14.28,3.5 U4.3
ATK0-RX  (via drill 0.2)
  Top 0.152: U4.5 12.93,4.78 v12.9,4.8 | U3.48 15.05,13.61 18.7,9.96 18.7,8.45 v18.1,7.85
  Bottom 0.152: v12.9,4.8 14.9,4.8 17.7,7.6 17.85,7.6 v18.1,7.85
ATK0-RXLED  (via drill 0.2)
  Top 0.152: U3.47 14.55,13.66 14.95,13.26 14.95,12.83 16.08,11.7 v16.08,11.67 | 5.2,10.9 R3.1 5.28,10.77 v6.04,10.77
  Bottom 0.152: v16.08,11.67 16.18,11.77 16.18,16.53 16.1,16.61 16.1,17.61 15.96,17.74 8.04,17.74 7.9,17.61 7.9,13.24 7.89,13.23 7.89,12.9 6.43,11.43 6.13,11.43 6.04,11.35 v6.04,10.77
ATK0-TX  (via drill 0.2)
  Top 0.152: U3.49 15.8,14.15 19.9,10.05 19.9,7.2 20.6,6.5 20.6,4.1 v19.2,2.7 | v9.9,2.7 9.8,2.8 8.38,2.8 U4.15
  Bottom 0.152: v19.2,2.7 v9.9,2.7
ATK0-TXLED  (via drill 0.2)
  Top 0.152: U3.46 14.05,13.72 14.64,13.13 14.64,12.7 15.47,11.88 15.47,11.49 15.73,11.22 15.73,10.78 15.7,10.75 15.7,10.6 16.05,10.25 16.17,10.25 17.08,9.34 v18,9.34 | R1.1 20.4,12.75 v20.4,12.5
  Bottom 0.152: v20.4,12.5 20.4,10.1 19.5,9.2 18.13,9.2 v18,9.34
ATK-CLKOUT  (via drill 0.2)
  Top 0.152: v8.2,7.45 8.35,7.3 U4.9 | v20.3,2 21.3,3 21.3,7.5 21.2,7.6 21.2,10.4 16.63,14.97 16.58,14.97 16.27,15.28 16.27,15.34 16.25,15.35 U3.50
  Bottom 0.152: v8.2,7.45 8.6,7.05 8.6,2.5 9.3,1.8 20.1,1.8 v20.3,2
BST
  Top 0.203: U1.10 14.85,35.65 15.1,35.9 C3.1
GND  (via drill 0.2, 0.35)
  Top 0.152: U3.44 13.05,13.4 C20.2 | S1.P$2 v21.2,39.2
  Top 0.203: 15.35,33.05 U1.TH 14.35,33.55 | 13.85,34.05 v14.1,34.3
  Top 0.254: U3.60 15.05,20.35 v14.7,20.7 | U3.52 15.35,16.35 14.7,17 13.05,15.35 U3.44 | U3.24 7.65,18.85 v7.9,18.6 | U3.14 8.55,21.35 8.05,20.85 | 8.05,20.85 v7.9,20.7 | 15.35,33.05 U1.4 | 14.35,33.55 U1.15 | U1.14 13.85,34.05 | U3.34 8.05,20.85
  other vias: 20,17 24.7,20.5 22,17.8 24.8,18.5 23.1,16.8 20.4,15.5 24.2,15.8 21.7,14 22.6,12.5 25.1,14.7 23.2,11 25.7,13.3 25.7,11.3 26.8,10.4 29.4,18.4 28.7,16.1 29.3,14 28.8,11.5 31.2,18.8 31.2,21.5 28.7,20.9 28.7,20 11.4,3.9 20.6,9.5 19.8,11 21.3,12.5 20.5,18.6 23.2,21.1 14.7,18.6 11.3,18.6 11.3,20.7 21.7,22.5 28.6,23.1 25.6,28.8 8.6,25.3 30,23.3 30,25.1 30.7,26.9 31.4,29.1 30.2,31.3 27.5,32.1 17.9,31.4 10,28.4 11.2,27.2 10.2,26.2 17.6,20.7 20.3,21.1 3.2,2.4 14.6,33.8 15.1,33.3 14.1,33.3 15.1,34.3 20,33.4 20,32.4 18.9,31.4 21,31.4 22,31.4 20,31.4 8,32 8,31.2 8.6,27.4 15.2,39.4 15.8,39.4 15.8,38.2 15.2,38.2 15.2,38.8 15.8,38.8 0.8,24 0.8,26 0.8,28 0.8,30 0.8,32 0.8,34 0.8,36 0.8,38 0.8,25 0.8,27 0.8,29 0.8,31 0.8,33 0.8,35 0.8,37 0.8,39 1.9,13.6 18.8,27.8 16.4,27.8 22.5,27.8 7.3,7.5 3.2,0.7 2.05,8.3 2.7,15.05 4.15,22.75 3.6,20.8 11.55,31.45 22.05,26.3 34.25,32.25 31.2,16.4 31.25,13.7 34,10.35 29.5,8 34,3.5 12.6,24.9 6.55,27.35 6.5,25.05 6.7,23.8 14.05,7.55 18,23.05 16.15,23.85 14.2,25.8 6.4,13.5 13.5,10.7 9.45,11.1 11.35,10.7 19.3,14 16.8,15.5 16.8,14 10,1.1 5.7,9 3.9,12.7 7,3.4 5.5,3 7,1.6 0.8,2.9 5.4,0.8 9.4,18.6 13,18.6 13.5,20.7 9.4,20.7 2,21.1 2.4,16.6 24.3,4.6 17.8,3.4 27,1 12.2,26.2 23,1 7.35,11.4 19.1,7.9 18.3,12.5 17.9,33.4 18.9,33.4 18.9,32.4 17.9,32.4 34.35,28.95 32.05,29.85 34.35,25.95 34.35,24.15 34.35,22.45 34.35,20.05 34.35,17.55 34.35,14.45 31.55,10.25
  pour Top (rank 6): -1.5,42 36.5,42 36.5,-1 -1.5,-1
  pour Bottom (rank 6): -2.5,43 37.5,43 37.5,-2 -2.5,-2
  pour Route2 (rank 6): -3,43.5 38,43.5 38,-2.5 -3,-2.5
  pour Route15 (rank 6): -3.5,44 38.5,44 38.5,-3 -3.5,-3
  pour Top (no thermals): 14.8,40.8 14.8,37.9 16.2,37.9 16.2,40.8
  pour Top (no thermals): 3.5,40.5 3.5,23.7 3,23.2 -0.4,23.2 -0.4,40.5
  pour Top (rank 5, no thermals): 17,34.3 27.5,34.3 28.5,33.3 28.5,32.4 28.2,32.1 28,31.9 24.4,31.9 22.8,31.9 21.3,30.4 17,30.4 16.8,30.6 16.8,33.5 16.8,34.1
N$1
  Top 0.152: U3.58 17.55,19.35 18.25,18.65 Y1.1
N$2
  Top 0.152: U3.59 17.55,19.85 18.25,20.55 Y1.3
N$8  (via drill 0.2)
  Top 0.152: R7.2 15.75,2.85 15.72,2.83 U4.2 13.47,2.83 v12.8,3.5
  Bottom 0.152: v12.8,3.5 12.3,4 12.3,5.2 12.9,5.8 13.5,5.8 15.17,7.47 15.17,9.77 14.55,10.38 14.55,12.36 15.57,13.37 J100.P$8
N$9
  Top 0.152: D5.2 2.4,5.65 R6.2
N$10
  Top 0.152: D4.2 2.4,9.15 R4.2
N$11
  Top 0.152: D3.2 2.4,12.65 R2.2
N$12  (via drill 0.2)
  Top 0.152: R7.1 14.68,2.18 U4.1 14.03,2.4 13.15,2.4 12.18,3.37 v12.04,3.37
  Bottom 0.152: v12.04,3.37 12.1,3.43 12.1,3.77 11.99,3.88 11.99,5.33 12.77,6.11 13.37,6.11 14.86,7.6 14.86,9.64 14.25,10.25 14.25,14.96 J100.P$7
N$13  (via drill 0.2)
  Top 0.152: v10.1,3.5 10,3.5 9.97,3.48 U4.14
  Bottom 0.152: v10.1,3.5 11.69,5.09 11.69,5.46 13.51,7.28 13.51,9.19 13.53,9.22 13.53,9.72 13.53,9.73 12.77,10.48 12.77,12.48 13.53,13.23 J100.P$6
N$14  (via drill 0.2)
  Top 0.152: U4.13 8.38,4.1 v9.6,4.1
  Bottom 0.152: v9.6,4.1 9.95,4.1 9.98,4.14 10.3,4.14 11.39,5.22 11.39,5.58 13.21,7.4 13.21,8.5 12.47,9.24 12.47,15.22 J100.P$5
N$15  (via drill 0.2)
  Top 0.152: R5.2 15.9,6.3 15.68,6.08 U4.7 12.78,6.08 v11.75,7.1
  Bottom 0.152: v11.75,7.1 11.47,7.39 11.47,9.07 11.53,9.14 11.53,9.72 11.22,10.04 11.07,10.04 10.61,10.5 10.61,12.41 11.49,13.29 J100.P$4
N$16  (via drill 0.2)
  Top 0.152: R5.1 15.9,5.3 15.7,5.5 14.32,5.5 U4.6 13.47,5.43 13.13,5.77 12.6,5.77 12.23,6.14 11.61,6.14 v11.14,6.6
  Bottom 0.152: v11.14,6.6 11.16,6.63 11.16,8.49 10.47,9.18 10.47,9.72 10.3,9.89 10.3,15.09 J100.P$3
N$17  (via drill 0.2)
  Top 0.152: v10.1,5.6 9.93,5.43 U4.11
  Bottom 0.152: v10.1,5.6 10.2,5.7 10.2,7 8.75,8.45 8.75,9.49 8.5,9.73 8.5,12.31 9.45,13.25 J100.P$2
N$18  (via drill 0.2)
  Top 0.152: U4.10 9.5,6.08 v9.61,6.19
  Bottom 0.152: v9.61,6.19 9.89,6.47 9.89,6.88 8.45,8.33 8.45,9.36 8.2,9.6 8.2,13.1 8.43,13.33 J100.P$1
PDI/DATA
  Top 0.152: U3.56 17.6,18.35 18.13,17.82 20.1,17.82 20.25,17.67 20.95,17.67 21.44,18.16 21.44,21.3 20.04,22.7 J101.1
PWMAHS  (via drill 0.2)
  Top 0.152: U3.17 5.9,22.35 v5.8,22.25 | v24.05,26.84 24.32,26.84 24.9,27.42 27.07,27.42 U$100.P$58
  Route15 0.152: v5.8,22.25 6.02,22.03 6.18,22.03 6.41,21.8 7.33,21.8 7.45,21.91 19.45,21.91 24.05,26.52 v24.05,26.84
PWMALS  (via drill 0.2)
  Top 0.152: v6.16,22.97 6.3,23.1 U3.16 | U$100.P$59 26.25,28.1 25.87,27.72 24.77,27.72 24.64,27.6 v24.32,27.6
  Route15 0.152: v6.16,22.97 6.91,22.22 19.32,22.22 23.5,26.4 23.5,27.04 23.83,27.37 24.1,27.37 v24.32,27.6
PWMBHS  (via drill 0.2)
  Top 0.152: U3.19 6,21.35 v5.84,21.19 | U$100.P$56 25.7,26.3 v25.12,26.89
  Route15 0.152: v5.84,21.19 7.59,21.19 7.7,21.3 19.7,21.3 25.12,26.72 v25.12,26.89
PWMBLS  (via drill 0.2)
  Top 0.152: U3.18 6.15,21.85 6.02,21.72 5.61,21.72 5.56,21.67 v5.24,21.67 | U$100.P$57 25.99,26.9 v25.92,26.84
  Route15 0.152: v5.24,21.67 5.56,21.67 5.61,21.72 6.05,21.72 6.28,21.5 7.46,21.5 7.57,21.61 19.57,21.61 24.58,26.62 24.58,27.11 24.9,27.42 25.34,27.42 v25.92,26.84
PWMCHS  (via drill 0.2)
  Top 0.152: U3.21 5.48,20.35 5.41,20.42 4.65,20.42 v4.5,20.26 | U$100.P$54 25.34,25.1 v25.1,24.87
  Route15 0.152: v4.5,20.26 4.82,20.26 4.97,20.42 5.41,20.42 6.02,19.81 20.25,19.81 24.46,24.03 24.46,24.15 24.95,24.64 25.07,24.64 25.1,24.67 v25.1,24.87
PWMCLS  (via drill 0.2)
  Top 0.152: U$100.P$55 25.47,25.7 v25.4,25.64 | v4.38,21.65 5.31,20.72 5.54,20.72 5.6,20.66 6.05,20.66 6.25,20.85 U3.20
  Route15 0.152: v25.4,25.64 25.16,25.4 24.88,25.4 24.57,25.09 24.57,24.69 24.16,24.28 24.16,24.16 20.12,20.12 6.14,20.12 5.54,20.72 5.31,20.72 v4.38,21.65
PWMDHS  (via drill 0.2)
  Top 0.152: U3.23 4.65,19.35 v4.5,19.5 | U$100.P$52 25.4,23.9 v25.3,23.8
  Route15 0.152: v4.5,19.5 4.8,19.2 20.5,19.2 25.1,23.8 v25.3,23.8
PWMDLS  (via drill 0.2)
  Top 0.152: U$100.P$53 25.81,24.5 v25.74,24.44 | v5.19,19.89 5.42,19.66 5.8,19.66 6,19.85 U3.22
  Route15 0.152: v25.74,24.44 25.64,24.34 25.08,24.34 24.77,24.02 24.77,23.9 20.37,19.51 5.57,19.51 v5.19,19.89
PWMEHS  (via drill 0.2)
  Top 0.152: U3.31 5.86,15.35 5.77,15.26 5.19,15.26 4.97,15.05 4,15.05 3.6,14.65 v3.5,14.65 | U$100.P$16 30.83,19.7 v30.76,19.77
  Route15 0.152: v30.76,19.77 30.76,19.84 30.6,20 30.13,20 27.73,17.6 25.13,17.6 22.38,14.85 21.33,14.85 21.02,14.55 3.6,14.55 v3.5,14.65
PWMELS  (via drill 0.2)
  Top 0.152: U$100.P$15 v31.3,20.3 | U3.30 6.75,15.8 5.88,15.8 5.65,15.57 5.06,15.57 4.9,15.4 v3.55,15.4
  Route15 0.152: v31.3,20.3 30,20.3 27.6,17.9 25,17.9 22.25,15.15 21.2,15.15 20.9,14.85 4.1,14.85 v3.55,15.4
RST  (via drill 0.2)
  Top 0.152: U3.57 17.53,18.85 18.25,18.13 20.23,18.13 20.38,17.97 20.82,17.97 21.13,18.28 21.13,21.17 19.4,22.9 19.4,23.77 19.05,24.12 19.05,25.43 18.95,25.53 | 18.95,25.53 15.95,25.53 J101.5 | 18.95,25.53 20.36,25.53 v21.9,27.06
  Bottom 0.152: v21.9,27.06 22.11,27.27 23.24,27.27 24.1,28.13 26.67,28.13 27.1,27.7 27.1,23.5 29.4,21.2 30.75,21.2 30.98,20.97 31.42,20.97 33,22.55 33,31.8 32.2,32.6 28.4,32.6 23.32,37.68 S1.P$4
  other vias: 21.2,37.68
RXLED  (via drill 0.2)
  Bottom 0.152: J100.GRNN 5.02,12.93 R3.2
  other vias: 5.2,12.75
STLCLK  (via drill 0.2)
  Top 0.152: v16.8,23.15 15.1,23.15 U3.1 | R4.1 2.5,7.98 3.33,8.81 3.33,10.9 3.73,11.3 v4.1,11.3
  Bottom 0.152: v4.1,11.3 5.45,11.3 5.88,11.74 6.3,11.74 7.59,13.03 7.59,17.73 7.91,18.05 9.84,18.05 14.95,23.15 v16.8,23.15
STLERR  (via drill 0.2)
  Top 0.152: v13.86,23.91 14.09,23.68 14.28,23.68 14.55,23.42 U3.2 | v4.7,11.84 3.48,11.84 R2.1
  Bottom 0.152: v13.86,23.91 13.86,22.5 10.57,19.2 7.75,19.2 7.29,18.74 7.29,13.15 6.17,12.04 5.75,12.04 5.32,11.61 4.93,11.61 v4.7,11.84
TW1/SCL  (via drill 0.2)
  Top 0.152: U3.37 9.55,13.6 9.36,13.42 9.36,12.13 8.61,11.37 8.61,10.53 8.9,10.24 9.07,10.24 10.1,9.2 v10.1,8.75 | v25.63,16.45 25.89,16.7 U$100.P$40
  Route15 0.152: v10.1,8.75 10.1,10.3 12.89,13.1 22.73,13.1 25,15.37 25.32,15.37 25.63,15.68 v25.63,16.45
TW1/SDA  (via drill 0.2)
  Top 0.152: U$100.P$42 25.9,17.9 25.1,17.1 v25.1,15.9 | U3.36 9.06,12.26 8.3,11.5 8.3,10.4 8.8,9.9 8.97,9.9 9.33,9.54 9.33,9.13 v9.37,9.1
  Route15 0.152: v25.1,15.9 22.6,13.4 12.7,13.4 9.79,10.5 9.79,9.52 v9.37,9.1
TXLED  (via drill 0.2)
  Top 0.152: v17.7,15.5 18.63,14.58 R1.2
  Bottom 0.152: J100.YLWN v17.71,15.51 v17.7,15.5
UART1/RX  (via drill 0.2)
  Top 0.152: U3.38 10.05,13.55 10.09,13.51 10.09,10.31 v11,9.4 | v31.2,17.9 U$100.P$19
  Route15 0.152: v11,9.4 11,9.5 13.4,11.9 14.47,11.9 14.47,11.91 15.13,11.91 15.73,12.5 16.42,12.5 17.09,11.84 23.04,11.84 28.9,17.7 30.2,17.7 30.4,17.9 v31.2,17.9
UART1/TX  (via drill 0.2)
  Top 0.152: U$100.P$20 30.73,17.3 v30.66,17.37 | v12,8.85 12,9.2 10.4,10.8 10.4,13.45 10.55,13.6 U3.39
  Route15 0.152: v30.66,17.37 29,17.37 23.16,11.54 16.96,11.54 16.3,12.2 15.86,12.2 15.54,11.89 15.54,11.85 15.3,11.6 14.6,11.6 13.55,11.6 12,10.05 v12,8.85
USART1/CSN  (via drill 0.2)
  Top 0.152: U$100.P$49 25.4,22.1 25.1,21.8 v24.8,21.8 | v3.02,17.34 3.32,17.64 4.96,17.64 5.06,17.74 6.69,17.74 U3.26
  Route15 0.152: v24.8,21.8 20.9,17.9 5.9,17.9 5.84,17.84 3.52,17.84 v3.02,17.34
USART1/RX  (via drill 0.2)
  Top 0.152: U$100.P$46 25.57,20.3 v25.29,20.02 | v4.1,16.4 4.55,16.85 U3.28
  Route15 0.152: v25.29,20.02 25.01,20.02 21.4,16.4 v4.1,16.4
USART1/SCK  (via drill 0.2)
  Top 0.152: v3.78,17.11 3.92,17.25 6.7,17.25 U3.27 | v25.2,21.15 25.56,21.5 U$100.P$48
  Route15 0.152: v3.78,17.11 4.21,17.54 5.96,17.54 6.03,17.6 21.03,17.6 24.57,21.15 v25.2,21.15
USART1/TX  (via drill 0.2)
  Top 0.152: U3.29 6,16.35 5.52,15.87 3.87,15.87 v3.34,16.4 | v25.3,19.26 25.75,19.7 U$100.P$45
  Route15 0.152: v3.34,16.4 3.87,15.87 5.52,15.87 5.75,16.1 21.53,16.1 24.69,19.26 v25.3,19.26
USART2/CSN  (via drill 0.2)
  Top 0.152: U3.40 11.05,13.45 11.23,13.27 11.23,11.67 13,9.9 v13,9.5 | v29,15.2 28.4,15.2 28.1,14.9 U$100.P$37
  Route15 0.152: v13,9.5 13.2,9.5 14.1,10.4 23.6,10.4 28.4,15.2 v29,15.2
USART2/RX  (via drill 0.2)
  Top 0.152: v15.7,9.1 15.7,9.3 12.29,12.71 12.29,13.51 12.05,13.75 U3.42 | v28.9,13.1 U$100.P$34
  Route15 0.152: v28.9,13.1 28.3,13.1 24,8.8 17.17,8.8 16.67,9.3 16.23,9.3 16.03,9.1 v15.7,9.1
USART2/SCK  (via drill 0.2)
  Top 0.152: U3.41 11.55,11.81 14.03,9.32 v14.09,9.32 | U$100.P$36 28.25,14.3 v28.54,14.59
  Route15 0.152: v14.09,9.32 14.09,9.92 14.27,10.1 23.73,10.1 28.22,14.59 v28.54,14.59
USART2/TX  (via drill 0.2)
  Top 0.152: U3.43 12.6,14.05 12.6,12.84 15.8,9.64 15.92,9.64 16.75,8.81 v16.75,8.47 | U$100.P$33 28.43,12.5 v28.44,12.49
  Route15 0.152: v28.44,12.49 28.12,12.49 24.13,8.5 16.75,8.5 v16.75,8.47
USBDM  (via drill 0.2)
  Top 0.152: U3.32 6.2,14.85 5.05,13.7 3.05,13.7 1.8,14.95 1.8,19 2.14,19.35 v2.39,19.35
  Bottom 0.152: v2.39,19.35 2.94,19.89 2.94,36.24 3.5,36.81 6.2,36.81 6.35,36.65 X100.D-
USBDP  (via drill 0.2)
  Top 0.152: U3.33 5.88,14.1 5.18,13.4 2.92,13.4 1.5,14.83 1.5,19.2 v2.4,20.1
  Bottom 0.152: v2.4,20.1 2.63,20.34 2.63,36.37 3.38,37.11 6.59,37.11 7,36.7 X100.D+
VCC
  pour Top (no thermals): 35.5,33 28.5,33 27.5,34 17.3,34 17.3,32 16.7,31.4 14.2,31.4 14.2,37.5 16.6,37.5 16.6,40.5 35.5,40.5
VSW
  pour Top (rank 2, no thermals): 14,31.4 14,37.7 16.4,37.7 16.4,40.5 9.6,40.5 9.6,34.4 9.8,34.2 11.3,34.2 11.9,33.6 11.9,32.1 12.6,31.4

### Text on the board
tPlace: VCC | a thick fog indeed / its opaque shimmer falls / once we go through it | ERR | LOOP | GND | PWR
bPlace: RESET | VCC | PDI | motherboard-xmega / V0.11 | ERR | LOOP | GND | PWR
